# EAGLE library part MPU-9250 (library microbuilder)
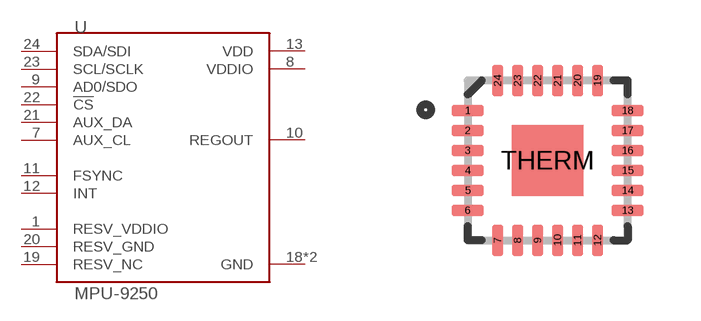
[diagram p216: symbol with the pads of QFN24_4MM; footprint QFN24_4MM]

Designator prefix -

## MPU-9250  [QFN24_4MM]
1  RESV_VDDIO
7  AUX_CL
8  VDDIO
9  AD0/SDO
10  REGOUT
11  FSYNC
12  INT
13  VDD
18  GND
19  RESV_NC
20  RESV_GND
21  AUX_DA
22  !CS
23  SCL/SCLK
24  SDA/SDI
THERM  GND

## Footprint QFN24_4MM (pad centres in mm)
smd 0.8 x 0.28: 1 -2,1.25; 2 -2,0.75; 3 -2,0.25; 4 -2,-0.25; 5 -2,-0.75; 6 -2,-1.25; 13 2,-1.25; 14 2,-0.75; 15 2,-0.25; 16 2,0.25; 17 2,0.75; 18 2,1.25
smd 0.28 x 0.8: 7 -1.25,-2; 8 -0.75,-2; 9 -0.25,-2; 10 0.25,-2; 11 0.75,-2; 12 1.25,-2; 19 1.25,2; 20 0.75,2; 21 0.25,2; 22 -0.25,2; 23 -0.75,2; 24 -1.25,2
smd 1.778 x 1.778: THERM 0,0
